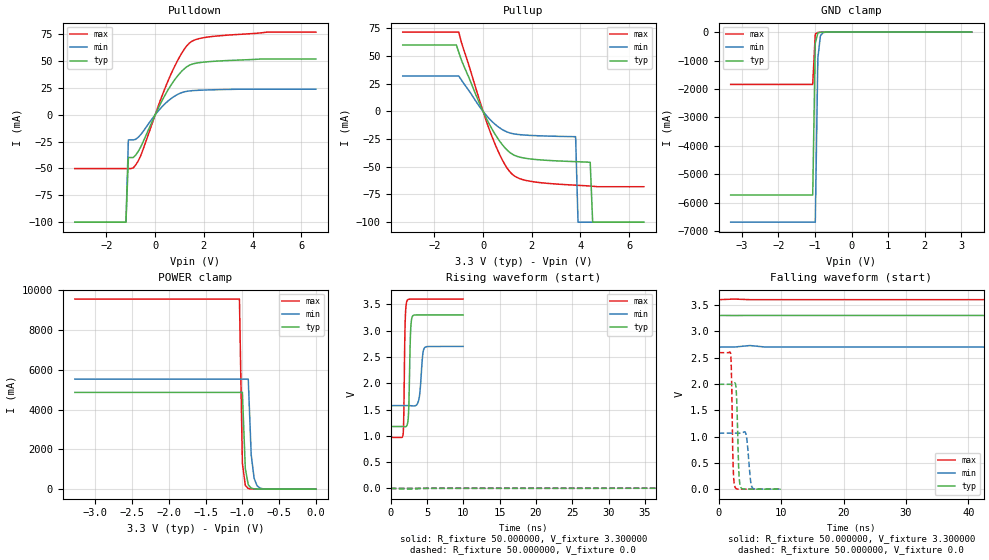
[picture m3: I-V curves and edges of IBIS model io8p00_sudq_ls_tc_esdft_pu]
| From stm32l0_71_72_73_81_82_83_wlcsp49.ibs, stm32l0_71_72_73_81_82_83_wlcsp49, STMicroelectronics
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|   Model io8p00_sudq_ls_tc_esdft_pu
[Model]  io8p00_sudq_ls_tc_esdft_pu
Model_type I/O
Polarity   Non-Inverting
Enable   Active-Low
Vinl =   0.990000V
Vinh =   2.310000V
Vmeas =  1.650000V
Cref =   50.000000pF
Rref =   100.000000M
Vref =   0.0V
C_comp   2.248300pF   2.207300pF   2.311900pF
[Temperature Range]   25.000000   0.125000k   -40.000000
[Pullup Reference]   3.300000V   2.700000V   3.600000V
[Pulldown Reference]   0.0V   0.0V   0.0V
[POWER Clamp Reference]   3.300000V   2.700000V   3.600000V
[GND Clamp Reference]   0.0V   0.0V   0.0V
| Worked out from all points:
|   slope of the pulldown table from 0 to 0.495 V, typ, clamps not added: 22.6 ohm
|   slope of the pullup table from 0 to 0.495 V, typ, clamps not added: 23.9 ohm
|   GND clamp passes 1 mA (typ) near -0.64 V on its own axis
|   POWER clamp passes 1 mA (typ) near -0.63 V on its own axis
|   rising waveform, R_fixture 50.000000, V_fixture 3.300000: 20-80 % time 209ps typ, 363ps min, 164ps max; typ from 1.18 V to 3.3 V
|   rising waveform, R_fixture 50.000000, V_fixture 0.0: 20-80 % time 210ns typ, 428ns min, 103ns max; typ from 0.001 V to 1.99 V
|   falling waveform, R_fixture 50.000000, V_fixture 3.300000: 20-80 % time 193ns typ, 383ns min, 106ns max; typ from 3.3 V to 1.18 V
|   falling waveform, R_fixture 50.000000, V_fixture 0.0: 20-80 % time 289ps typ, 458ps min, 227ps max; typ from 1.99 V to 0.001 V
[Pulldown]
|Voltage   I(typ)   I(min)   I(max)
-3.3V     -100mA     -100mA     -50.11mA
-1.2V     -100mA     -100mA     -50.11mA
-1.1V     -39.8mA    -23.37mA   -50.11mA
-900mV    -39.8mA    -23.37mA   -49.43mA
-600mV    -30.26mA   -18.59mA   -38.38mA
500mV     22.11mA    12.28mA    30.06mA
900mV     35.58mA    18.71mA    49.62mA
1.3V      44.73mA    21.88mA    64.23mA
1.7V      48.13mA    22.72mA    70.3mA
2.4V      49.79mA    23.3mA     73.03mA
4.6V      51.9mA     23.82mA    77mA
6.6V      51.9mA     23.82mA    77mA
[Pullup]
|Voltage   I(typ)   I(min)   I(max)
-3.3V     60mA       32mA       71.6mA
-1.1V     60mA       32mA       71.6mA
-1V       53.5mA     32mA       71.6mA
-100mV    4.893mA    2.926mA    6.861mA
400mV     -17.21mA   -9.813mA   -24.69mA
900mV     -32.92mA   -17.72mA   -48.15mA
1.3V      -39.75mA   -20.4mA    -58.47mA
3.8V      -45.36mA   -22.8mA    -66.6mA
3.9V      -45.44mA   -100mA     -66.72mA
4.4V      -46mA      -100mA     -67.4mA
4.5V      -100mA     -100mA     -67.56mA
6.6V      -100mA     -100mA     -68mA
[GND_clamp]
|Voltage   I(typ)   I(min)   I(max)
-3.3V     -5.732A    -6.688A    -1.842A
-1.06V    -5.732A    -6.688A    -1.842A
-990mV    -389.4mA   -6.688A    -68.34mA
-920mV    -32.57mA   -918.2mA   -10.72mA
-850mV    -6.763mA   -131mA     -6.509mA
-780mV    -3.471mA   -21mA      -4.208mA
3.28V     0A         0A         0A
[POWER_clamp]
|Voltage   I(typ)   I(min)   I(max)
-3.28V    4.87A      5.538A     9.569A
-1.04V    4.87A      5.538A     9.569A
-1V       4.87A      5.538A     1.315A
-960mV    1.032A     5.538A     186.5mA
-920mV    222.2mA    5.538A     31.65mA
-880mV    50.75mA    1.734A     9.59mA
-840mV    13.94mA    544.9mA    5.676mA
-800mV    5.568mA    172.7mA    4.284mA
-760mV    3.243mA    55.85mA    3.306mA
-680mV    1.609mA    7mA        1.749mA
0V        0A         0A         0A
[Ramp]
| variable   typ   min   max
dV/dt_r  1.19497/0.20981u   0.60760/0.42875u   1.55546/0.10328u
dV/dt_f  1.27200/0.19299u   0.63480/0.38411u   1.57747/0.10595u
R_load = 50.000000
[Rising Waveform]
R_fixture= 50.000000
V_fixture= 3.300000
V_fixture_min= 2.700000
V_fixture_max= 3.600000
|time   V(typ)   V(min)   V(max)
0s        1.178V     1.575V     970.9mV
1.702ns   1.178V     1.575V     1.021V
2.002ns   1.174V     1.575V     3.193V
2.262ns   1.209V     1.575V     3.572V
2.482ns   1.52V      1.575V     3.596V
2.743ns   2.991V     1.574V     3.599V
2.963ns   3.262V     1.571V     3.599V
3.864ns   3.299V     1.683V     3.6V
4.645ns   3.3V       2.672V     3.6V
9.97ns    3.3V       2.7V       3.6V
[Rising Waveform]
R_fixture= 50.000000
V_fixture= 0.0
V_fixture_min= 0.0
V_fixture_max= 0.0
|time   V(typ)   V(min)   V(max)
0s        1.075mV    1.827mV    669.2uV
57.56ns   4.11mV     4.6mV      107.5mV
115.1ns   93.61mV    4.812mV    1.009V
175.2ns   416.6mV    6.554mV    1.919V
217.7ns   705.6mV    15.99mV    2.294V
257.8ns   982.8mV    38.56mV    2.461V
377.9ns   1.58V      172.3mV    2.575V
545.5ns   1.897V     458.2mV    2.591V
865.9ns   1.986V     883mV      2.593V
1.246us   1.993V     1.064V     2.593V
[Falling Waveform]
R_fixture= 50.000000
V_fixture= 3.300000
V_fixture_min= 2.700000
V_fixture_max= 3.600000
|time   V(typ)   V(min)   V(max)
0s        3.3V       2.7V       3.6V
82.58ns   3.3V       2.7V       3.496V
145.1ns   3.213V     2.7V       2.59V
210.2ns   2.866V     2.697V     1.63V
247.7ns   2.611V     2.687V     1.252V
282.8ns   2.362V     2.669V     1.095V
397.9ns   1.62V      2.546V     998.5mV
510.5ns   1.323V     2.357V     979.7mV
860.9ns   1.194V     1.759V     971.3mV
1.246us   1.178V     1.575V     970.9mV
[Falling Waveform]
R_fixture= 50.000000
V_fixture= 0.0
V_fixture_min= 0.0
V_fixture_max= 0.0
|time   V(typ)   V(min)   V(max)
0s        1.993V     1.064V     2.593V
1.922ns   1.993V     1.064V     2.57V
2.322ns   1.994V     1.064V     449.7mV
2.643ns   2.017V     1.064V     37.19mV
2.883ns   1.726V     1.064V     6.699mV
3.263ns   277.6mV    1.064V     1.12mV
3.524ns   41.27mV    1.064V     843.1uV
4.404ns   1.246mV    1.031V     738uV
5.385ns   1.122mV    30.16mV    702.7uV
9.97ns    1.075mV    1.827mV    669.2uV
